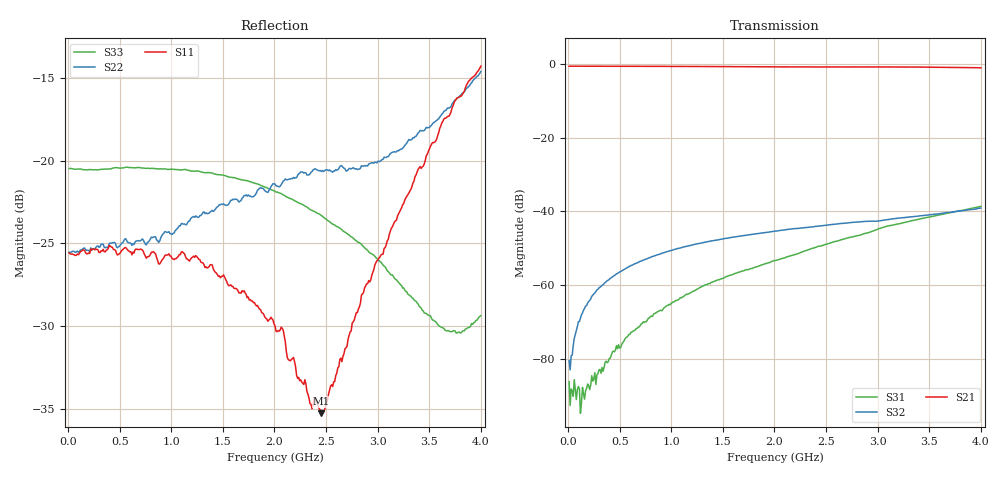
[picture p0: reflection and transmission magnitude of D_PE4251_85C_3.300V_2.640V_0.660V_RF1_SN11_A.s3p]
! Device ID: PE4251_SoldCshunt_081809
! Dir: c:\Test Bench Repositories\Bench_Software_CVI_Version_8\trunk\PSC 4Port_VNA Bench\datalog\4250\TEST\PE4251_SoldCshunt_081809\85C\3p300000\RF1
! Serial: 11
! Insertion: A
! Temp: 85C
! VDD: 3.300
! Control_Hi: 80.000
! Control_Lo: 20.000
! Logic State: RF1
! Port 1: RFC
! Port 2: RF1
! Port 3: RF2
! V1 = 0.66
! V2 = 2.64
! V3 = 0.66
! IDD: 5.548440e-05
! FILE NAME
! DATE 08/18/09  20:17
! CORRECTED  DATA
#  Hz  S  RI  R  50.00
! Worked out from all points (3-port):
!   401 points, 10 MHz to 4 GHz, reference 50 ohm
!   strongest paths, dB at 10 MHz, 1.008 GHz, 2.005 GHz, 3.002 GHz, 4 GHz:
!     S21: -0.6, -0.7, -0.8, -0.8, -1.1
!     S32: -80.4, -50.5, -45.3, -42.6, -39.1
!     S31: -86.2, -64.8, -53.4, -44.8, -38.6
!   lowest |S11| = -35.3 dB at 2.454 GHz (marker M1), VSWR 1.04, Z = 49.9 - j1.72 ohm
!   |S11| at or under -10 dB: start of sweep to end of sweep
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1e7  0.0526 0.000158  0.9306 -0.00359  2.34e-05 -1.1e-05
     0.9307 -0.00468  0.0528 0.000175  4.26e-05 -5.12e-05
     4.12e-05 -2.69e-05  9.28e-05 -2.17e-05  0.0947 -0.00036
1.0975e8  0.0524 -0.000534  0.9309 -0.0382  2.6e-05 -1.31e-05
          0.9309 -0.0382  0.0531 -0.000396  4.09e-05 0.000326
          3.07e-05 -2.48e-05  5.81e-05 0.000316  0.0943 -0.00244
1.79575e8  0.0523 -0.00119  0.9295 -0.0621  1.66e-05 -3.53e-05
           0.9289 -0.0619  0.0536 -0.00128  5.85e-05 0.000553
           3.54e-06 -3.98e-05  6.97e-05 0.000526  0.0938 -0.00421
3.79075e8  0.0536 -0.004  0.9216 -0.127  -5.43e-05 -6.95e-05
           0.9212 -0.127  0.0544 -0.00322  0.000104 0.00115
           -6.17e-05 -6.41e-05  0.000105 0.00115  0.0938 -0.00952
5.287e8  0.0535 -0.0051  0.9126 -0.1756  -0.000146 -9.42e-05
         0.9124 -0.175  0.0563 -0.00371  0.000157 0.00159
         -0.000138 -9.33e-05  0.000162 0.00159  0.0942 -0.0128
1.14715e9  0.0472 -0.0178  0.8481 -0.3673  -0.000742 -6.74e-05
           0.8489 -0.3664  0.0608 -0.0199  0.000553 0.00332
           -0.000752 -7.28e-05  0.000547 0.00333  0.0908 -0.0238
2.005e9  0.0261 -0.0179  0.703 -0.5826  -0.00216 0.000153
         0.7033 -0.5825  0.0717 -0.0457  0.000988 0.0053
         -0.00214 0.000142  0.00098 0.00532  0.0748 -0.0307
2.453875e9  -0.000417 -0.0172  0.6106 -0.6736  -0.00341 0.000244
            0.6101 -0.6739  0.0621 -0.069  0.00104 0.00629
            -0.00341 0.000246  0.00103 0.0063  0.0604 -0.0316
3.650875e9  -0.1125 -0.0739  0.284 -0.8552  -0.00887 0.00275
            0.2857 -0.8535  -0.0615 -0.1277  -0.000113 0.00954
            -0.00888 0.00273  -0.000132 0.00957  0.00512 -0.0303
4e9  -0.176 -0.08  0.1592 -0.8725  -0.0109 0.00437
     0.1578 -0.8696  -0.1364 -0.1267  -0.000738 0.0111
     -0.0109 0.00436  -0.000772 0.0111  -0.0158 -0.0301
